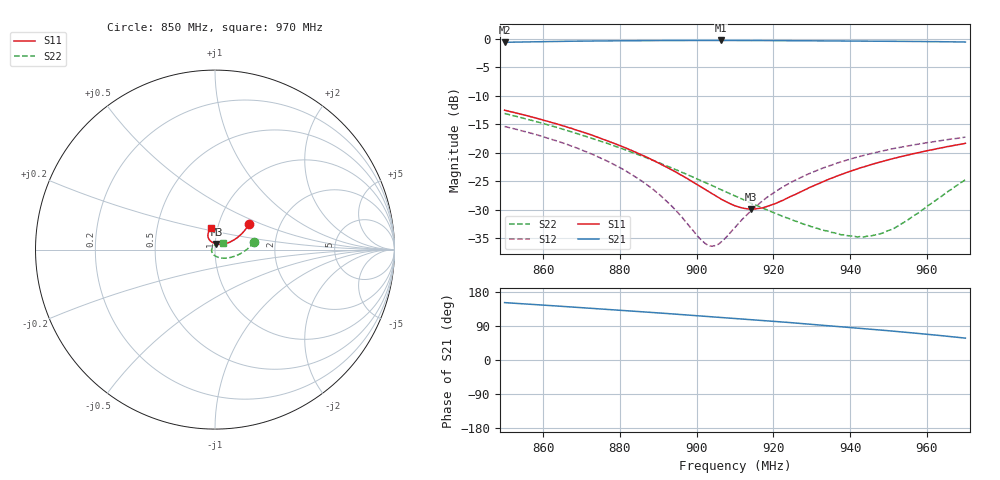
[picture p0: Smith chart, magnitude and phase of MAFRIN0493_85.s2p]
!Part Number:  MAFRIN0493
!Name:  MC
!Comments:  1
!Thu 09/Dec/2004  2:55:55 PM
!Temperature:  85
# MHZ  S  DB  R  50
!Freq  S11(dB)  S11(ang)  S21(dB)  S21(ang)  S12(dB)  S12(ang)  S22(dB)  S22(ang)
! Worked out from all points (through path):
!   201 points, 850 MHz to 970 MHz, reference 50 ohm
!   highest |S21| = -0.28 dB at 906.4 MHz (marker M1); lowest = -0.6 dB at 850 MHz (marker M2)
!   lowest |S11| = -29.9 dB at 914.2 MHz (marker M3), VSWR 1.07, Z = 50.7 + j3.15 ohm
!   |S11| at or under -10 dB: start of sweep to end of sweep
!   |S22| runs from -34.8 to -13.1 dB; largest |S21 - S12| = 1.1
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850  -12.51 36.9  -0.60 151.4  -15.37 102.2  -13.08 10.7
862  -14.62 31.8  -0.45 143.5  -17.55 91.0  -15.22 -0.7
870.4  -16.37 28.9  -0.40 137.9  -19.58 82.5  -16.92 -9.4
881.2  -19.05 26.8  -0.33 130.5  -23.02 69.9  -19.41 -22.2
886  -20.45 26.8  -0.31 127.1  -25.06 62.9  -20.62 -28.6
890.2  -21.81 27.4  -0.29 124.1  -27.23 55.2  -21.71 -35.1
893.8  -23.08 29.0  -0.29 121.5  -29.51 46.4  -22.71 -41.0
900.4  -25.65 35.0  -0.29 116.8  -34.71 15.4  -24.64 -52.9
902.2  -26.39 37.9  -0.29 115.5  -35.87 -0.0  -25.18 -56.6
904  -27.14 41.2  -0.28 114.1  -36.36 -18.9  -25.73 -60.5
906.4  -28.12 47.0  -0.28 112.4  -35.62 -45.0  -26.46 -65.8
910  -29.28 58.2  -0.29 109.7  -33.09 -73.6  -27.55 -74.7
914.2  -29.87 75.0  -0.30 106.5  -30.13 -91.9  -28.82 -86.1
917.2  -29.64 87.2  -0.31 104.2  -28.37 -100.3  -29.68 -95.2
921.4  -28.62 101.2  -0.31 101.0  -26.41 -108.6  -30.83 -108.6
930.4  -25.78 116.8  -0.34 93.8  -23.32 -121.1  -33.00 -142.3
937.6  -23.80 120.1  -0.36 88.0  -21.58 -128.8  -34.35 -174.3
941.8  -22.83 120.1  -0.38 84.5  -20.75 -132.9  -34.75 164.3
947.2  -21.71 118.3  -0.41 79.7  -19.83 -137.9  -34.30 132.8
950.2  -21.16 117.1  -0.42 77.0  -19.42 -140.4  -33.55 116.2
958  -19.91 111.7  -0.46 69.8  -18.43 -146.9  -30.43 78.0
970  -18.31 100.1  -0.55 57.8  -17.23 -155.6  -24.71 40.2
